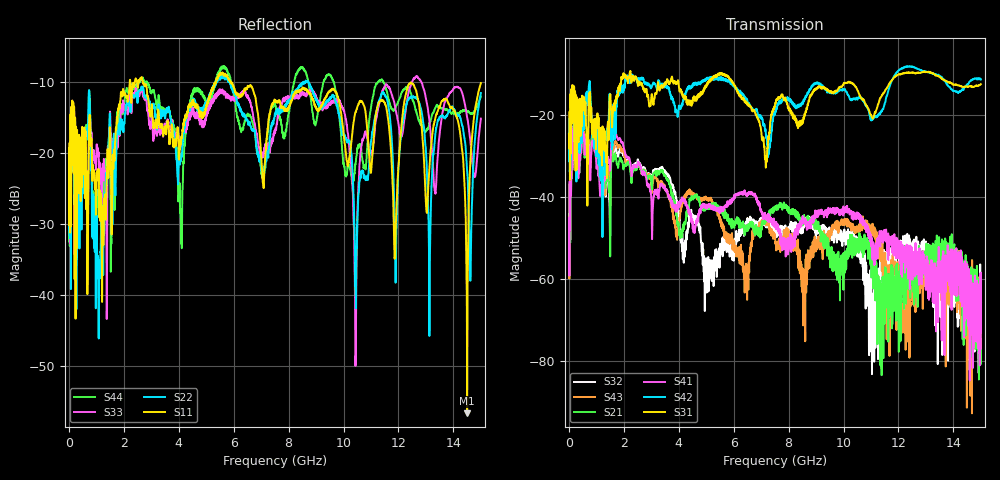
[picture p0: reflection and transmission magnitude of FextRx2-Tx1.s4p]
! FILE: N:\QM 2007\Prüfprotokolle\Highspeed\Konfektionierte Ltg\L45593-D106\D30\8216\0002\Fext\FextRx2-Tx1.s4p
# MHz S DB R 50.00
! FREQ  S11  S12  S13  S14
!  S21  S22  S23  S24
!  S31  S32  S33  S34
!  S41  S42  S43  S44
!  DB  ANG  DB  ANG  DB  ANG  DB  ANG
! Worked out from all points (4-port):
!   2999 points, 10 MHz to 15 GHz, reference 50 ohm
!   strongest paths, dB at 10 MHz, 3.755 GHz, 7.505 GHz, 11.26 GHz, 15 GHz:
!     S31: -24.6, -10.5, -17.4, -17.3, -12.4
!     S42: -24.4, -15.4, -19.7, -19.9, -11.2
!     S41: -45.0, -40.8, -46.8, -52.1, -76.9
!     S21: -49.0, -38.9, -42.9, -60.7, -65.6
!     S43: -48.4, -43.1, -49.3, -51.5, -66.2
!     S32: -44.1, -37.2, -47.7, -79.5, -60.5
!   lowest |S11| = -56.7 dB at 14.5 GHz (marker M1), VSWR 1.00, Z = 50 - j0.143 ohm
!   |S11| at or under -10 dB: start of sweep to 2.214 GHz; 2.696 GHz to 5.333 GHz (2.637 GHz wide, 65.7 % of centre); 5.923 GHz to end of sweep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
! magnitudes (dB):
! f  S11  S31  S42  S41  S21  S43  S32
! 10 MHz  -19.3  -24.6  -24.4  -45.0  -49.0  -48.4  -44.1
! 900 MHz  -22.3  -21.8  -23.3  -27.0  -25.3  -25.2  -24.7
! 9.795 GHz  -12.0  -13.6  -13.9  -43.2  -57.7  -46.7  -49.0
! 10.43 GHz  -14.2  -13.0  -16.1  -44.0  -50.9  -48.3  -51.2
! 12.47 GHz  -10.1  -9.5  -8.1  -52.1  -55.8  -64.0  -57.8
! 14.5 GHz  -56.7  -13.0  -12.5  -56.3  -57.4  -62.9  -68.8
! 15 GHz  -10.1  -12.4  -11.2  -76.9  -65.6  -66.2  -60.5
